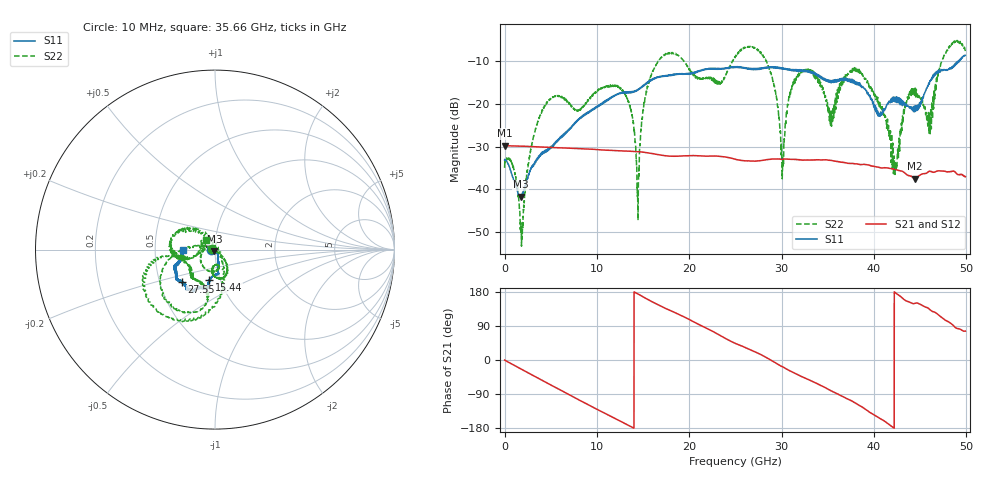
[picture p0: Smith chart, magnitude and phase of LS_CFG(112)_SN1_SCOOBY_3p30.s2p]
!Keysight Technologies,N5245B,MY58422026,A.13.80.08
!Date: Friday, March 20, 2020 00:02:20
!Correction: S11(Full 2 Port(1,2))
!S21(Full 2 Port(1,2))
!S12(Full 2 Port(1,2))
!S22(Full 2 Port(1,2))
!S2P File: Measurements: S11, S21, S12, S22:
# Hz S DB R 50.0
!freq dBS11 angS11 dBS21 angS21 dBS12 angS12 dBS22 angS22
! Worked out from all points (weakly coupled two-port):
!   4991 points, 10 MHz to 49.91 GHz, reference 50 ohm
!   highest |S21| = -29.71 dB at 10 MHz (marker M1); lowest = -37.5 dB at 44.42 GHz (marker M2)
!   lowest |S11| = -41.7 dB at 1.77 GHz (marker M3), VSWR 1.02, Z = 49.7 - j0.767 ohm
!   |S11| at or under -10 dB: start of sweep to 49.12 GHz; 49.16953 GHz to 49.22316 GHz (53.63 MHz wide, 0.109 % of centre)
!   |S22| runs from -53.3 to -5.1 dB; largest |S21 - S12| = 0.00032
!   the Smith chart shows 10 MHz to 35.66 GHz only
!   S11 on the Smith chart (normalised r, x): 10 MHz: 0.96, -0.01; 15.44 GHz: 0.89, -0.31; 27.55 GHz: 0.65, -0.25; 35.66 GHz: 0.69, +0.00
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1e7  -33.10 -172.9  -29.71 -0.1  -29.72 -0.3  -34.94 177.1
1.77e9  -41.67 -110.7  -29.85 -23.5  -29.85 -23.4  -48.81 -34.2
4.23e9  -31.54 -55.9  -30.07 -55.7  -30.08 -55.6  -20.88 -151.2
8.33e9  -23.20 -75.0  -30.45 -108.9  -30.45 -108.8  -21.02 -92.8
1.276e10  -17.39 -81.4  -30.98 -163.9  -30.98 -163.8  -16.76 -63.1
1.445e10  -16.71 -93.7  -31.14 174.2  -31.13 174.3  -46.31 -114.8
1.544e10  -15.17 -100.6  -31.41 160.8  -31.40 160.9  -16.41 174.3
1.665e10  -13.74 -100.4  -31.85 145.3  -31.84 145.4  -9.97 -157.3
2.496e10  -11.40 -125.8  -32.88 44.2  -32.86 44.5  -9.08 -167.9
2.755e10  -11.70 -135.7  -33.28 16.8  -33.27 17.1  -7.63 -110.2
2.914e10  -11.50 -141.7  -32.85 -4.7  -32.85 -4.4  -15.05 -72.6
3.011e10  -11.81 -145.5  -32.92 -17.7  -32.91 -17.4  -34.62 15.2
3.116e10  -12.00 -150.1  -32.96 -31.7  -32.96 -31.3  -15.62 140.2
3.328e10  -12.56 -159.8  -33.09 -56.0  -33.09 -55.6  -12.34 -175.2
3.566e10  -14.89 179.4  -33.30 -84.7  -33.24 -84.2  -22.00 129.8
3.816e10  -15.45 172.6  -34.02 -116.0  -33.97 -116.1  -11.57 -174.6
4.16e10  -19.46 101.3  -35.02 -169.3  -35.02 -169.3  -25.68 67.5
4.233e10  -18.66 101.4  -35.31 177.7  -35.33 177.7  -33.69 165.3
4.442e10  -21.82 52.7  -37.49 149.2  -37.50 149.6  -17.84 -11.1
4.6e10  -15.33 6.2  -35.73 134.3  -35.74 134.5  -24.52 112.1
4.771e10  -11.99 5.6  -35.75 105.5  -35.76 105.8  -8.16 -80.0
4.991e10  -8.58 -13.5  -36.99 76.2  -37.00 76.2  -7.38 -14.7
